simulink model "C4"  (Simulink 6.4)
settings: Solver=ode45  StartTime=0.0  StopTime=10.0  RelTol=1e-3
libraries: cstblocks x2

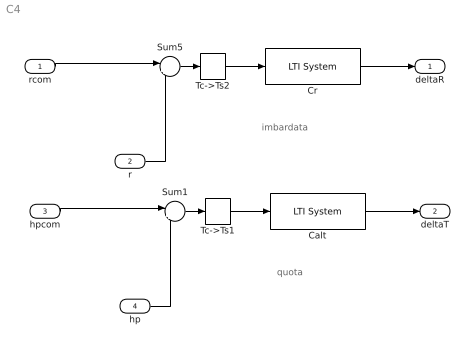
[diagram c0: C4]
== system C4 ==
  note: imbardata
  note: quota
  rcom : Inport
  r : Inport  Port=2
  hpcom : Inport  Port=3
  hp : Inport  Port=4
  Calt : cstblocks/LTI System  SystemSampleTime=-1  sys=C4altd  IC=[]
  Cr : cstblocks/LTI System  SystemSampleTime=-1  sys=C4rd  IC=[]
  Sum1 : Sum  Inputs=|+-
  Sum5 : Sum  Inputs=|+-
  Tc->Ts1 : RateTransition  Deterministic=off  OutPortSampleTime=Ts
  Tc->Ts2 : RateTransition  Deterministic=off  OutPortSampleTime=Ts
  deltaR : Outport
  deltaT : Outport  Port=2
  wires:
  Sum5/1 -> Tc->Ts2/1
  rcom/1 -> Sum5/1
  Tc->Ts2/1 -> Cr/1
  r/1 -> Sum5/2
  Cr/1 -> deltaR/1
  Sum1/1 -> Tc->Ts1/1
  hpcom/1 -> Sum1/1
  Tc->Ts1/1 -> Calt/1
  hp/1 -> Sum1/2
  Calt/1 -> deltaT/1
